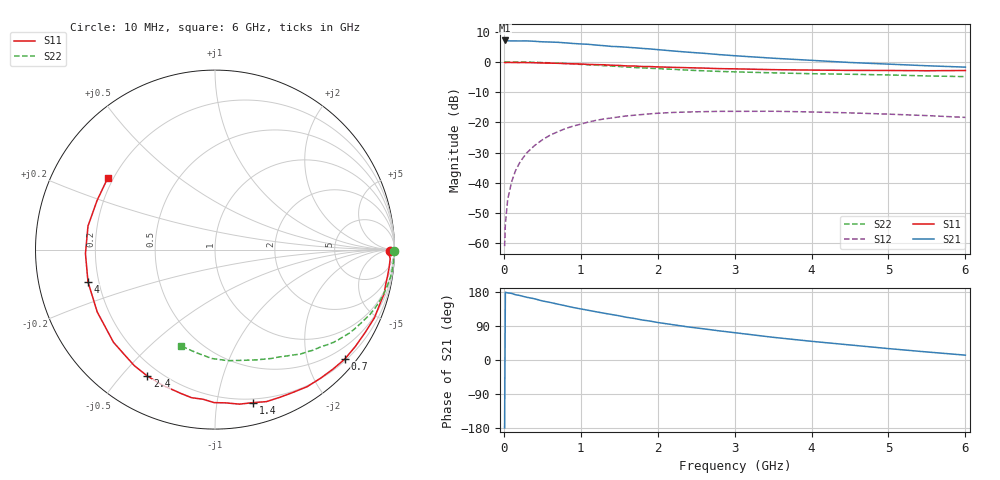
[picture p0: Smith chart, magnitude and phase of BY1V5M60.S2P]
! SIEMENS Small Signal Semiconductors
! BFY420
! Si NPN RF SIEGET Grounded Emitter Transistor in MICRO-X
! VCE = 1.5 V  IC = 0.6 mA
! Common Emitter S-Parameters:  October  1996
# GHz  S  MA  R  50
!  f  S11  S21  S12  S22
! GHz  MAG  ANG  MAG  ANG  MAG  ANG  MAG  ANG
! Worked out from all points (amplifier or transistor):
!   36 points, 10 MHz to 6 GHz, reference 50 ohm
!   highest |S21| = 7.1 dB at 10 MHz (marker M1)
!   |S21| within 3 dB of that: start of sweep to 1.987 GHz
!   unconditionally stable (mu >= 1): 4.718 GHz to end of sweep
!   at 250 MHz: K = 0.04, MSG = 19.3 dB, |S12| = -31.7 dB
!   at 1.4 GHz: K = 0.20, MSG = 11.8 dB, |S12| = -18.6 dB
!   at 6 GHz: K = 1.40, MAG = 4.6 dB, |S12| = -18.4 dB
!   S11 on the Smith chart (normalised r, x): 10 MHz: 73, -34; 700 MHz: 0.23, -2.72; 1.4 GHz: 0.17, -1.26; 2.4 GHz: 0.15, -0.59; 4 GHz: 0.16, -0.12; 6 GHz: 0.18, +0.29
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0.01  0.9778 -0.6  2.254 -179.2  0.0009 94.4  0.9997 -0.3
0.02  0.9683 -1.3  2.251 178.9  0.0021 82.6  0.9999 -0.6
0.05  0.9777 -3.0  2.225 177.1  0.0053 91.3  0.9992 -1.4
0.1  0.9752 -5.9  2.214 175.8  0.0103 86.7  0.9964 -3.0
0.15  0.9728 -8.6  2.216 172.3  0.0157 84.4  0.9964 -4.4
0.25  0.9743 -14.6  2.215 167.9  0.026 80.1  0.9936 -7.3
0.4  0.9664 -23.1  2.183 161.5  0.0414 75.5  0.9818 -11.7
0.5  0.9559 -28.7  2.141 155.9  0.0514 71.5  0.9725 -14.4
0.7  0.946 -40.1  2.101 147.5  0.0699 64.8  0.9501 -19.9
0.9  0.9268 -50.8  2.01 138.6  0.0867 57.3  0.9214 -24.9
1.1  0.9058 -61.8  1.947 131.1  0.1014 51.0  0.8936 -29.8
1.4  0.8785 -76.1  1.797 120.1  0.1181 42.1  0.851 -36.2
1.6  0.856 -86.0  1.742 112.5  0.1279 36.4  0.8199 -40.3
1.8  0.8363 -94.6  1.666 105.5  0.1347 31.6  0.7937 -43.7
2.2  0.8105 -110.9  1.511 93.1  0.1457 22.1  0.7519 -50.7
2.4  0.799 -118.1  1.441 87.2  0.1484 18.4  0.7279 -53.9
2.8  0.7718 -131.4  1.316 76.9  0.1519 11.3  0.694 -59.7
3.5  0.7425 -152.1  1.147 59.9  0.1525 1.1  0.6573 -69.1
4  0.7302 -165.7  1.058 49.3  0.1485 -4.7  0.6359 -76.0
4.5  0.7221 -178.2  0.975 39.7  0.1434 -9.7  0.6231 -83.3
5.5  0.7117 157.4  0.861 21.2  0.1293 -15.7  0.5846 -99.9
6  0.7184 146.3  0.817 12.8  0.1207 -16.5  0.5695 -109.2
